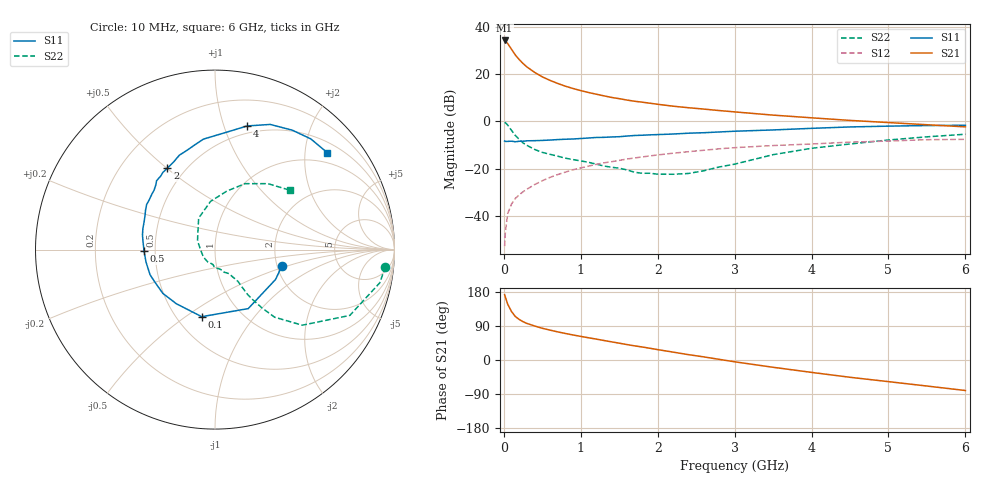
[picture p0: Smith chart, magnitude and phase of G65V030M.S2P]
! SIEMENS Small Signal Semiconductors
! BFG193
! Si NPN RF Bipolar Junction Transistor in SOT223
! VCE = 5 V  IC = 30 mA
! Common Emitter S-Parameters:  August  1996
# GHz  S  MA  R  50
!  f  S11  S21  S12  S22
! GHz  MAG  ANG  MAG  ANG  MAG  ANG  MAG  ANG
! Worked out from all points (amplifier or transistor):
!   36 points, 10 MHz to 6 GHz, reference 50 ohm
!   highest |S21| = 34.2 dB at 10 MHz (marker M1)
!   |S21| within 3 dB of that: start of sweep to 84.72 MHz
!   unconditionally stable (mu >= 1): 583.6 MHz to 2.47 GHz
!   at 250 MHz: K = 0.83, MSG = 27.1 dB, |S12| = -29.8 dB
!   at 1.4 GHz: K = 1.04, MAG = 12.3 dB, |S12| = -17.1 dB
!   at 6 GHz: K = 0.89, MSG = 2.6 dB, |S12| = -7.6 dB
!   S11 on the Smith chart (normalised r, x): 10 MHz: 2.13, -0.45; 100 MHz: 0.66, -0.58; 500 MHz: 0.43, -0.01; 2 GHz: 0.40, +0.50; 4 GHz: 0.43, +1.20; 6 GHz: 0.73, +2.50
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0.01  0.3844 -13.4  51.32 172.2  0.0023 90.9  0.9542 -5.7
0.02  0.3761 -26.3  49.99 166.0  0.0046 82.7  0.9365 -11.4
0.05  0.3773 -60.6  44.14 147.4  0.0112 73.9  0.836 -26.0
0.1  0.381 -101.2  33.35 127.8  0.0179 65.9  0.6434 -40.9
0.15  0.3707 -125.6  25.25 114.6  0.0236 62.1  0.5021 -48.6
0.2  0.3794 -140.0  20.23 107.0  0.028 63.6  0.4152 -51.2
0.25  0.3805 -151.2  16.68 101.0  0.0325 63.2  0.3501 -53.0
0.3  0.3881 -158.8  14.16 96.5  0.0368 64.9  0.311 -54.0
0.4  0.3906 -169.7  10.85 89.8  0.0461 64.8  0.2548 -54.2
0.5  0.3954 -178.9  8.734 83.7  0.0556 64.8  0.2208 -54.1
0.6  0.4025 174.4  7.355 78.9  0.0654 64.2  0.2011 -55.1
0.8  0.4187 163.6  5.539 70.0  0.0846 61.9  0.1667 -58.5
1.1  0.445 150.4  4.078 58.7  0.1131 57.7  0.1364 -67.7
1.6  0.4893 132.3  2.821 40.7  0.1596 47.6  0.0942 -92.9
2  0.5253 120.3  2.297 27.4  0.1949 39.0  0.0765 -132.1
2.2  0.5401 115.2  2.094 20.8  0.2123 34.6  0.0762 -149.2
2.8  0.5967 100.4  1.692 1.7  0.2629 20.9  0.1086 153.5
3.5  0.6585 84.1  1.356 -19.2  0.3082 4.0  0.1978 117.4
4  0.7119 75.4  1.189 -32.7  0.3327 -5.8  0.2696 95.3
4.5  0.7622 66.2  1.048 -45.6  0.3637 -15.9  0.3326 78.6
5.5  0.8158 49.1  0.849 -68.7  0.4102 -39.2  0.4713 51.2
6  0.8266 40.8  0.765 -80.5  0.4169 -52.7  0.5343 38.1
